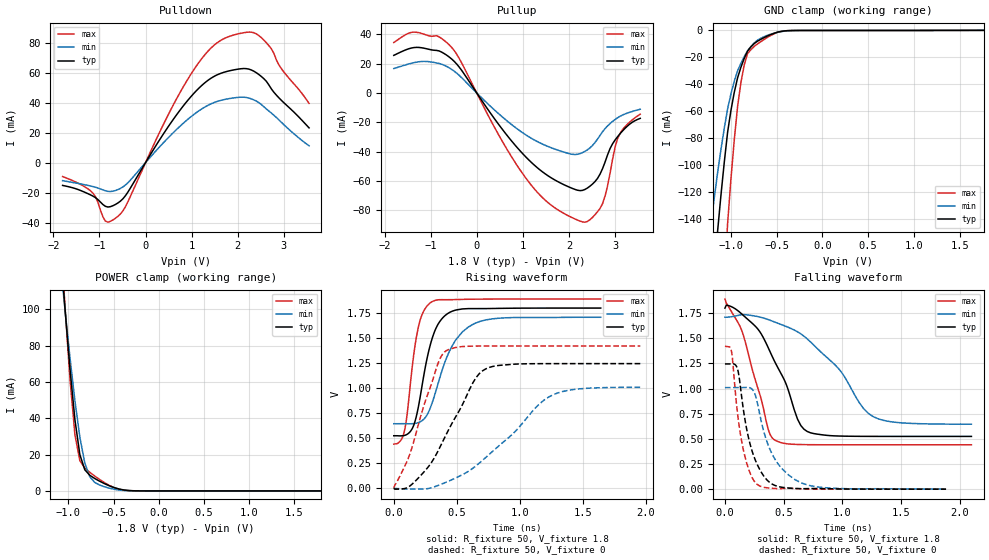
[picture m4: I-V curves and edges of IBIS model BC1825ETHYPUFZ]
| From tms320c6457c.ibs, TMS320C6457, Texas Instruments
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|   Model Cell BC1825ETHYPUFZ
[Model]   BC1825ETHYPUFZ
Model_type   I/O
Polarity   Non-Inverting
Enable   Active-Low
|BUFFER OPERATING IN WEAK PULL UP MODE WITH +/- 5% VDDS
Vinl =  0.63
Vinh =  1.17
Cref =  15pF
Rref =  100.00M
Vref =  0V
Vmeas =  0.9
C_comp   1.78948p   1.365653p   2.395095p
[Model Spec]
Vinl   0.63   0.5985   0.6615
Vinh   1.17   1.1115   1.2285
[Temperature Range]   25   125   -40
[Voltage Range]   1.8   1.71   1.89
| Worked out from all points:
|   slope of the pulldown table from 0 to 0.27 V, typ, clamps not added: 19.9 ohm
|   slope of the pullup table from 0 to 0.27 V, typ, clamps not added: 21.6 ohm
|   GND clamp passes 1 mA (typ) near -0.47 V on its own axis
|   POWER clamp passes 1 mA (typ) near -0.43 V on its own axis
|   rising waveform, R_fixture 50, V_fixture 1.8: 20-80 % time 128ps typ, 195ps min, 88.7ps max; typ from 0.525 V to 1.8 V
|   rising waveform, R_fixture 50, V_fixture 0: 20-80 % time 311ps typ, 499ps min, 213ps max; typ from 0.001 V to 1.25 V
|   falling waveform, R_fixture 50, V_fixture 1.8: 20-80 % time 285ps typ, 447ps min, 206ps max; typ from 1.8 V to 0.525 V
|   falling waveform, R_fixture 50, V_fixture 0: 20-80 % time 139ps typ, 201ps min, 103ps max; typ from 1.25 V to 0.001 V
[POWER_clamp]
|   voltage   I(typ)   I(min)   I(max)
-1.8V     660.1mA    532.8mA    797.4mA
-1.055V   111.6mA    108.6mA    115.6mA
-1.036V   99.87mA    99.38mA    101mA
-981.8mV  67.15mA    73.33mA    61.43mA
-927.3mV  39.17mA    49.6mA     30.9mA
-872.7mV  20mA       29.6mA     16.68mA
-818.2mV  11.65mA    15.37mA    12.61mA
-763.6mV  8.658mA    7.853mA    10.3mA
-709.1mV  6.873mA    4.723mA    8.231mA
-490.9mV  1.788mA    911.2uA    1.764mA
-327.3mV  204.2uA    86.16uA    166.5uA
1.8V      1.988nA    94.53nA    1.232nA
[Pulldown]
|   voltage   I(typ)   I(min)   I(max)
-1.8V     -15.25mA   -12.06mA   -9.369mA
-1.145V   -22.33mA   -15.98mA   -20.27mA
-872.7mV  -29.18mA   -18.79mA   -38.99mA
-600mV    -26.95mA   -18.03mA   -35.87mA
-436.4mV  -22.07mA   -14.95mA   -29.41mA
381.8mV   18.88mA    13.05mA    25.17mA
981.8mV   43.91mA    30.49mA    58.87mA
1.473V    57.25mA    39.86mA    77.92mA
1.909V    61.77mA    43.1mA     85.04mA
2.291V    61.77mA    42.49mA    86.97mA
2.509V    57.43mA    38.73mA    83.31mA
3.545V    23.12mA    11.18mA    39.46mA
[Pullup]
|   voltage   I(typ)   I(min)   I(max)
-1.8V     25.65mA    16.66mA    34.38mA
-1.364V   30.97mA    20.68mA    41.53mA
-872.7mV  29.05mA    20.49mA    39.06mA
-600mV    24.59mA    17.18mA    32.92mA
545.5mV   -24.38mA   -16.07mA   -32.47mA
1.091V    -44.45mA   -29.08mA   -59.11mA
1.636V    -58.24mA   -37.57mA   -76.98mA
2.291V    -66.39mA   -40.66mA   -87.87mA
2.673V    -55.32mA   -28.9mA    -78.7mA
2.782V    -47.12mA   -24.26mA   -70.3mA
3.055V    -29.77mA   -16.87mA   -31.03mA
3.545V    -17.27mA   -11.04mA   -14.43mA
[GND_clamp]
|   voltage   I(typ)   I(min)   I(max)
-1.8V     -735.6mA   -496.7mA   -1.298A
-1.218V   -207.8mA   -143.7mA   -387.5mA
-1.145V   -148.9mA   -105.5mA   -281.5mA
-1.036V   -75.64mA   -58.25mA   -143.6mA
-963.6mV  -46.07mA   -37.81mA   -81.49mA
-927.3mV  -35.26mA   -30.06mA   -56.52mA
-890.9mV  -27.42mA   -24.44mA   -38.8mA
-854.5mV  -20.8mA    -19.47mA   -25.71mA
-818.2mV  -15.41mA   -15.15mA   -17.23mA
-709.1mV  -8.029mA   -7.258mA   -10.07mA
-381.8mV  -245.5uA   -344.7uA   -239.3uA
1.764V    -4.378uA   4.316uA    -21.18uA
[Ramp]
| variable   typ   min   max
dV/dt_f   0.784409/0.2972378n  0.6544285/0.4657954n  0.8924378/0.2169803n
dV/dt_r  0.7520307/0.3138052n  0.6107526/0.5051814n  0.8580565/0.2148431n
R_load = 50
[Rising Waveform]
R_fixture = 50
V_fixture = 1.8
V_fixture_min = 1.71
V_fixture_max = 1.89
|   time   V(typ)   V(min)   V(max)
0s        525.4mV    645.5mV    442.2mV
54ps      524.1mV    645.7mV    476.8mV
88ps      529.7mV    645.7mV    591.7mV
158ps     628.3mV    646.8mV    1.329V
216ps     959.2mV    668.9mV    1.706V
292ps     1.441V     809.5mV    1.854V
362ps     1.659V     1.089V     1.883V
462ps     1.768V     1.418V     1.884V
642ps     1.795V     1.646V     1.889V
1.644ns   1.8V       1.708V     1.89V
[Rising Waveform]
R_fixture = 50
V_fixture = 0
V_fixture_min = 0
V_fixture_max = 0
|   time   V(typ)   V(min)   V(max)
0s        1.371mV    987.8uV    1.668mV
116ps     13.43mV    -6.728mV   302.7mV
184ps     89.09mV    -7.386mV   584.2mV
348ps     364.6mV    27.28mV    1.236V
418ps     541.9mV    62.75mV    1.375V
654ps     1.106V     225.9mV    1.42V
760ps     1.208V     341.6mV    1.421V
1.266ns   1.245V     934.7mV    1.421V
1.474ns   1.246V     993.3mV    1.421V
1.958ns   1.246V     1.009V     1.421V
[Falling Waveform]
R_fixture = 50
V_fixture = 1.8
V_fixture_min = 1.71
V_fixture_max = 1.89
|   time   V(typ)   V(min)   V(max)
0s        1.8V       1.71V      1.89V
140ps     1.745V     1.735V     1.586V
364ps     1.418V     1.688V     614.2mV
426ps     1.263V     1.661V     487.9mV
526ps     1.029V     1.616V     452.5mV
618ps     696.8mV    1.565V     445.6mV
728ps     561.5mV    1.465V     443.2mV
976ps     529.1mV    1.187V     442.3mV
1.262ns   525.8mV    722.2mV    442.2mV
2.098ns   525.4mV    647.2mV    442.2mV
[Falling Waveform]
R_fixture = 50
V_fixture = 0
V_fixture_min = 0
V_fixture_max = 0
|   time   V(typ)   V(min)   V(max)
0s        1.246V     1.011V     1.421V
58ps      1.247V     1.011V     1.355V
108ps     1.192V     1.011V     746.9mV
180ps     628.7mV    1.012V     282mV
242ps     341.7mV    978.8mV    94.18mV
280ps     233.8mV    837.3mV    44.34mV
344ps     110.9mV    520.3mV    17.26mV
420ps     41.22mV    310.7mV    8.327mV
658ps     5.835mV    59.68mV    5.349mV
1.882ns   1.386mV    2.715mV    1.669mV
